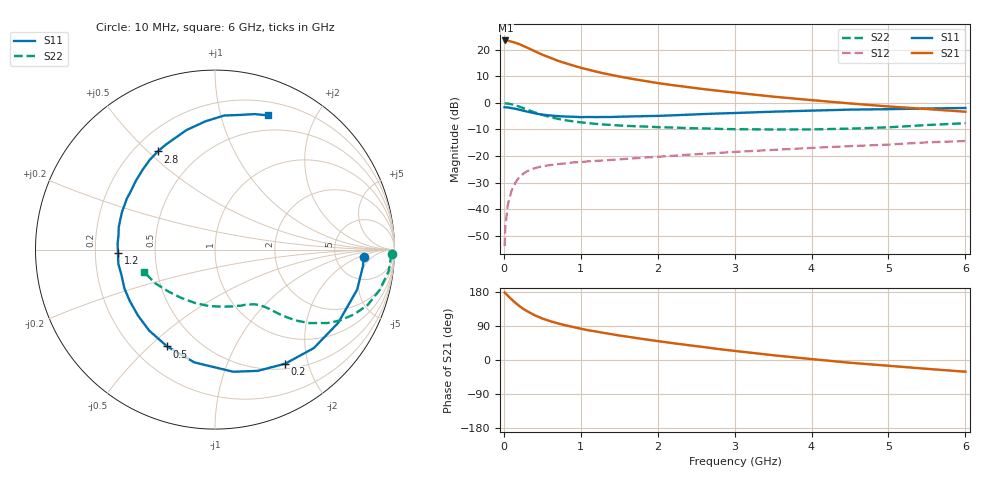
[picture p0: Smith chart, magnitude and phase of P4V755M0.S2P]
! SIEMENS Small Signal Semiconductors
! BFP182
! Si NPN RF Bipolar Junction Transistor in SOT143
! VCE = 0.75 V  IC = 5 mA
! Common Emitter S-Parameters:  March  1996
# GHz  S  MA  R  50
!  f  S11  S21  S12  S22
! GHz  MAG  ANG  MAG  ANG  MAG  ANG  MAG  ANG
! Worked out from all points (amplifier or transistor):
!   36 points, 10 MHz to 6 GHz, reference 50 ohm
!   highest |S21| = 23.6 dB at 20 MHz (marker M1)
!   |S21| within 3 dB of that: start of sweep to 324.8 MHz
!   unconditionally stable (mu >= 1): 1.397 GHz to end of sweep
!   at 250 MHz: K = 0.23, MSG = 24.1 dB, |S12| = -26.7 dB
!   at 1.4 GHz: K = 1.00, MAG = 15.8 dB, |S12| = -21.5 dB
!   at 6 GHz: K = 1.07, MAG = 3.9 dB, |S12| = -14.3 dB
!   S11 on the Smith chart (normalised r, x): 10 MHz: 10, -3; 200 MHz: 0.57, -1.64; 500 MHz: 0.34, -0.57; 1.2 GHz: 0.30, -0.02; 2.8 GHz: 0.29, +0.54; 6 GHz: 0.33, +1.42
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0.01  0.8301 -3.0  14.97 178.3  0.002 88.7  0.9849 -1.4
0.02  0.8293 -6.5  15.05 176.4  0.0047 89.4  0.9802 -2.9
0.05  0.8228 -15.7  14.89 169.9  0.0117 83.8  0.9752 -7.0
0.1  0.7985 -30.7  14.32 160.2  0.0223 72.9  0.9447 -13.8
0.15  0.7773 -44.9  13.61 151.0  0.0315 67.2  0.9043 -20.0
0.2  0.7463 -58.4  12.85 142.7  0.0397 60.5  0.8544 -25.0
0.25  0.7164 -70.6  11.9 135.3  0.0461 55.2  0.8002 -29.6
0.3  0.6881 -81.5  11.08 129.2  0.0514 50.6  0.7492 -33.1
0.4  0.6389 -100.4  9.464 118.2  0.0589 44.0  0.665 -38.0
0.5  0.6018 -116.3  8.123 109.5  0.0643 39.4  0.5958 -41.4
0.6  0.5816 -129.0  7.144 102.6  0.0674 36.1  0.5424 -43.6
0.7  0.565 -139.4  6.253 96.8  0.0703 33.9  0.5032 -45.2
0.9  0.5494 -156.6  5.078 87.1  0.0757 31.3  0.4497 -47.4
1.1  0.5443 -171.6  4.241 78.4  0.0795 29.9  0.4159 -49.5
1.2  0.541 -178.0  3.896 75.1  0.081 29.1  0.4029 -50.7
1.7  0.5592 157.8  2.792 58.7  0.0905 28.7  0.3644 -56.8
2.2  0.5846 138.9  2.16 44.4  0.1011 28.0  0.3444 -65.2
2.8  0.6329 120.2  1.687 28.7  0.1147 26.4  0.3244 -77.9
3.5  0.6844 103.5  1.316 12.6  0.1304 23.2  0.3162 -96.1
4.5  0.7488 86.1  0.979 -7.3  0.1536 18.0  0.328 -124.6
5.5  0.7862 73.8  0.768 -23.3  0.1808 12.1  0.3832 -150.9
6  0.8043 68.4  0.683 -30.9  0.1917 7.7  0.4154 -162.8
